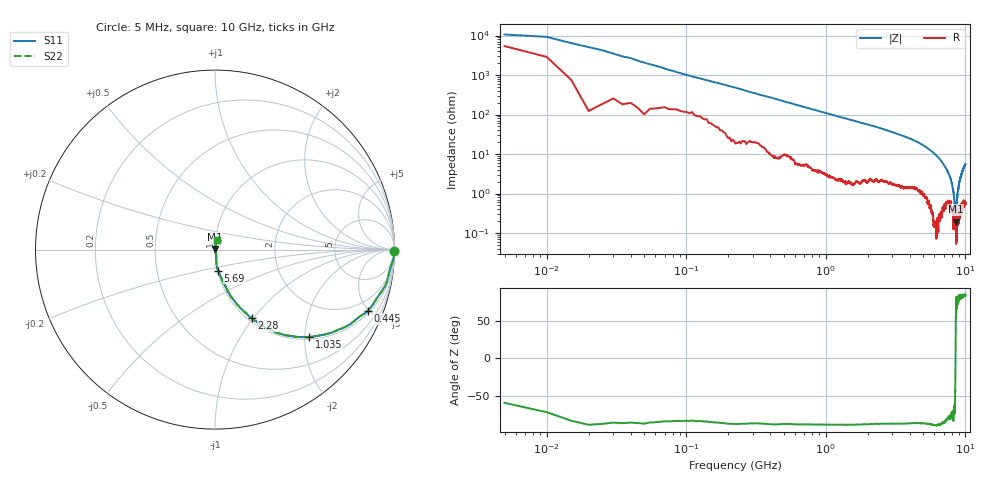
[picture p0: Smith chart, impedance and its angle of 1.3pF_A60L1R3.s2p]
! Amotech Co.,Ltd.
! http://www.amotech.co.kr/
! Part Number: A60L1R3
! These Parameters are Measured in Series Mode Connection
! Operation Temp=25[degC], DC Bias Voltage=0[V]
! Freq. Start=5[MHz] Stop=10[GHz], 2000[Steps]
! Date: Monday, July 14, 2020, 09:47:17
# GHZ S RI R 50.000000
!Freq.(Hz) S11(Real) S11(Imag) S21(Real) S21(Imag) S12(Real) S12(Imag) S22(Real) S22(Imag)
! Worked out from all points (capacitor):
!   2000 points, 5 MHz to 10 GHz, reference 50 ohm
!   read as one part in series: C = 1.57 pF near 55 MHz
!   lowest |Z| = 195 mohm at 8.52 GHz (marker M1)
!   series resonance near 8.493 GHz, so ESL is about 220 pH
!   S11 on the Smith chart (normalised r, x): 5 MHz: open; 445 MHz: 1.15, -4.91; 1.035 GHz: 1.05, -2.11; 2.28 GHz: 1.05, -0.98; 5.69 GHz: 1.01, -0.24; 10 GHz: 1.01, +0.11
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0.005  0.9952 -0.00801  0.0048 0.00801  0.0048 0.00801  0.9952 -0.00801
0.075  0.9872 -0.0722  0.0128 0.0722  0.0128 0.0722  0.9872 -0.0722
0.135  0.9712 -0.1248  0.0288 0.1248  0.0288 0.1248  0.9712 -0.1248
0.27  0.9312 -0.2317  0.0688 0.2317  0.0688 0.2317  0.9312 -0.2317
0.445  0.8504 -0.3414  0.1496 0.3414  0.1496 0.3414  0.8504 -0.3414
1.035  0.5251 -0.4865  0.4749 0.4865  0.4749 0.4865  0.5251 -0.4865
1.675  0.3121 -0.4485  0.6879 0.4485  0.6879 0.4485  0.3121 -0.4485
2.28  0.2043 -0.3805  0.7957 0.3805  0.7957 0.3805  0.2043 -0.3805
3.34  0.1013 -0.2769  0.8987 0.2769  0.8987 0.2769  0.1013 -0.2769
5.005  0.035 -0.1582  0.965 0.1582  0.965 0.1582  0.035 -0.1582
5.69  0.0181 -0.1167  0.9819 0.1167  0.9819 0.1167  0.0181 -0.1167
6.67  0.00799 -0.0676  0.992 0.0676  0.992 0.0676  0.00799 -0.0676
7.855  0.0058 -0.0222  0.9942 0.0222  0.9942 0.0222  0.0058 -0.0222
8.215  0.00173 -0.0106  0.9983 0.0106  0.9983 0.0106  0.00173 -0.0106
8.335  0.00197 -0.00502  0.998 0.00502  0.998 0.00502  0.00197 -0.00502
8.47  0.00192 -0.000819  0.9981 0.000819  0.9981 0.000819  0.00192 -0.000819
8.52  0.00142 0.00134  0.9986 -0.00134  0.9986 -0.00134  0.00142 0.00134
8.605  0.00121 0.00296  0.9988 -0.00296  0.9988 -0.00296  0.00121 0.00296
8.72  0.00248 0.00769  0.9975 -0.00769  0.9975 -0.00769  0.00248 0.00769
9.03  0.00337 0.0184  0.9966 -0.0184  0.9966 -0.0184  0.00337 0.0184
9.455  0.00501 0.0335  0.995 -0.0335  0.995 -0.0335  0.00501 0.0335
10  0.00842 0.0547  0.9916 -0.0547  0.9916 -0.0547  0.00842 0.0547
